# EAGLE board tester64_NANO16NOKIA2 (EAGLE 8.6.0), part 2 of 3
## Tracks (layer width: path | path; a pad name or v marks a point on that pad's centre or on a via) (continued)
+5V  (via drill 0.7, 0.7 pad 0.25) (continued)
  Top 0.61: U5.18 196.69,77.44 198.38,79.12 204,79.12 208.12,79.12 v209,79.25 | C7.2 U6.15 200.5,104.5 200,105 197.5,105 196.75,104.25 196.75,102.91 U6.18 | C7.2 209.48,102.85 v209.5,102.88 | U7.9 193.91,117.22 197.75,113.38 v206.88,113.38 | U7.18 196.44,130.94 196.5,131 199.12,131 | 199.12,131 203.75,131 206.75,131 v206.88,131.12 | U7.16 198.99,130.86 199.12,131 | U8.9 194.03,143.97 | U8.15 206.85,155.86 v207,156 | C7.2 | U6.9 194.16,92.09 196.98,89.26 v209.13,89.26 | v25,135.75 41.5,135.75 | 41.5,135.75 45.6,135.75 R86.2 | v41.25,138.25 41.25,136 41.5,135.75 | v29.75,108.75 29.75,109.75 31.5,111.5 34.24,111.5 C2.2 34.37,111.5 v38.5,111.5 39.5,112.5 R71.2 | v25.25,77 27.73,79.47 C6.2 29.02,79.5 v34.12,79.5 R55.2 | U5.9 194.16,63.09 v194.62,62.62 | R55.2 R54.2 R53.2 R52.2 R51.2 R50.2 R49.2 43.25,70.97 43.25,70 41.85,68.6 R48.2 R47.2 R46.2 R45.2 R44.2 R43.2 R42.2 R41.2 R40.2 | R55.2 R56.2 R57.2 R58.2 R59.2 R60.2 R61.2 R62.2 R63.2 R64.2 43.23,100.38 R65.2 R66.2 R67.2 R68.2 R69.2 R70.2 R71.2 | R33.2 R34.2 R35.2 R36.2 R37.2 R38.2 R39.2 R40.2 | R71.2 R72.2 R73.2 R74.2 R75.2 R76.2 R77.2 R78.2 R79.2 R80.2 R81.2 R82.2 R83.2 R84.2 R85.2 R86.2 | R86.2 R87.2 R88.2 R89.2 R90.2 R91.2 R92.2 R93.2 R94.2 R95.2 R96.2 v43.88,152 | v40.5,55.88 41.73,55.88 R40.2 | v215.5,89.25 212.25,89.25
  Top 0.813: v207,141.5 195.38,141.5 194.25,142.62 194.25,143.97 C4.2 | 199.45,46.25 R2.2 | U11.4 118.63,62.75 C44.+ 161,62.75 177.5,46.25 199.45,46.25 | U13.3 209.3,40.76 ARD1.J2.4 209.41,42.34 205.5,46.25 199.45,46.25 | 212.25,89.25 209.14,89.25 v209.13,89.26
  Bottom 0.406: U4.9 41.16,138.34 v41.25,138.25 | U1.18 U1.17 27.61,107.5 26.5,107.5 26,107 26,105.5 26.51,105 U1.15 | U2.18 21.93,49.43 21.62,49.12 21.62,46.88 | 21.62,46.88 21.62,46.12 22.25,45.5 22.9,45.5 U2.15 | U2.16 21.64,46.89 21.62,46.88 | 219.88,89.12 219.75,89.25
  Bottom 0.5: 36,55.88 33.62,53.5 33.62,52.75 32.84,51.97 U2.9 30.28,51.97 v30.5,52 | U2.18 24.93,49.43 v25.25,49.88
  Bottom 0.61: v207,156 v207,141.5 207,131.25 v206.88,131.12 v206.88,113.38 206.88,106 209.38,103.5 209.38,103 v209.5,102.88 209.38,102.88 208.66,102.16 208.66,90.28 209,89.94 v209.13,89.26 209,89.51 v209,79.25 209,72.12 203,66.12 203,62.62 | v25,135.75 25.75,135.75 25.8,135.81 U4.18 U4.17 U4.16 | U1.9 38.34,111.34 v38.5,111.5 | U1.18 29.7,108.81 v29.75,108.75 | U3.9 34.09,79.47 v34.12,79.5 | v25.25,77 23.09,77 U3.18 U3.17 | ARD1.J2.4 209.41,45.84 204.75,50.5 204.75,53.62 203,55.38 203,62.62 | v194.62,62.62 203,62.62 | 36,55.88 v40.5,55.88 | 220.75,80.5 220.75,88.25 219.88,89.12 | 219.75,89.25 v215.5,89.25
  Bottom 0.813: v43.88,152 43.88,170.5 56,182.62 203.38,182.62 206.88,179.12 206.88,156.12 v207,156 | 220.75,80.5 221.66,79.59 J22.3 J22.1 J22.2
A0
  Top 0.406: R103.2 R104.1 123.7,55.7 129,61 160,61 175.5,45.5 175.5,45.25 176,44.75 185.21,44.75 ARD1.J2.12
D0
  Top 0.61: SW6.2 150.75,43 161.5,32.25 161.5,21.25 164.5,18.25 208.75,18.25 214.5,24 ARD1.J1.2
  Bottom 0.61: SW6.2 SW6.1
D2  (via drill 0.7)
  Top 0.406: R106.1 85.25,64.5 v85.5,64.75
  Top 0.61: v85.5,68.75 159.25,68.75 v175.5,52.5
  Bottom 0.406: 85.5,65.25 v85.5,64.75 v85.5,68.75
  Bottom 0.61: v175.5,52.5 175.5,39.5 186.5,28.5 204,28.5 ARD1.J1.5
D11
  Top 0.61: SW3.2 SW3.1
  Bottom 0.406: SW3.1 176.05,15.55 184,23.5 ARD1.J1.14
D12
  Top 0.406: ARD1.J1.15 181.47,26.53 176.5,31.5 173.18,31.5 SW2.2
  Top 0.61: SW2.2 SW2.1
D13
  Top 0.406: SW1.1 176.8,35.8 181,40 181,40.4 ARD1.J2.15
  Top 0.61: SW1.2 SW1.1
DC.1
  Bottom 0.61: DIS1.J1.3 195.83,14.83 199,18 199,18.83 R138.1
DIN.1
  Bottom 0.61: DIS1.J1.4 198.37,14.62 202,18.25 R139.1
DSUB  (via drill 0.7)
  Top 0.406: v223.5,55.5 215.25,55.5 v215,55.75 | ARD1.J1.12 189.09,30.16 v189,30.25
  Bottom 0.406: J22.4 217.09,79.59 215,77.5 v215,55.75 | v189,30.25 222,30.25 223.75,32 223.75,55.25 v223.5,55.5
GND  (via drill 0.7, 0.7 pad 0.25)
  Top 0.406: C3.1 203.12,128.98 202.62,128.48 | v39.25,137 34.51,137 C1.1 | C8.1 203.62,77.88 203.75,78 | v34.62,50.75 35.5,50.75 35.62,50.62 36.12,50.62 36.38,50.38 36.25,50.25
  Top 0.5: C5.1 23.73,48.02 25.38,46.38
  Top 0.61: U6.10 195.43,92.2 197,90.62 v209.75,90.62 | v209.75,100.88 203.12,100.88 | 203.12,100.88 199.5,100.88 | 199.5,100.88 198.5,100.88 198,101.38 198,102.82 U6.17 | U6.16 199.24,101.14 199.5,100.88 | v210.12,78 203.75,78 199,78 197.97,76.97 U5.17 U5.16 U5.15 | v209.25,128.5 209.23,128.48 202.62,128.48 U7.15 200.25,127.25 199.62,126.62 198.38,126.62 197.72,127.28 U7.17 | U7.10 195.18,117.58 198,114.75 v209.25,114.75 | U8.10 195.3,144.68 C4.1 | C7.1 203.38,101.12 203.12,100.88 | C25.2 C26.2 C27.2 C28.2 C29.2 C30.2 C31.2 C32.2 | C33.2 C34.2 C35.2 C36.2 C37.2 C38.2 C39.2 C40.2 193.42,89.78 195.2,87.99 | v29.75,106.25 30,106.25 33.5,109.75 34.29,109.75 C2.1 34.54,109.5 v39,109.5 | v34.25,77.75 29.02,77.75 | 29.02,77.75 C6.1 | 29.02,77.75 28.5,77.75 v25.25,74.5 | R104.2 101.5,50.99 SW6.3 | C17.2 C18.2 C19.2 C20.2 C21.2 C22.2 C23.2 192.25,60.77 | 192.25,60.77 C24.2 | 192.28,60.75 192.25,60.77 | v30.5,50.62 29.5,50.62 v25.25,46.38
  Top 0.813: v209.25,142.88 197.1,142.88 C4.1 | C25.2 209.06,106.72 v209.25,106.53 | C1.1 23.63,137.13 23.25,136.75 | 23.25,131.5 v23.25,131.75 23.25,130.25 19.5,126.5 19.5,106.25 30,106.25 | ARD1.J1.4 209.3,25.74 U13.1 214.03,32.72 v214.25,32.5 | C44.- 125.5,67.5 112.75,67.5 110.95,65.7 U11.1 99.78,65.53 99.75,65.5 | Q2.2 71.55,53.3 | SW1.4 SW1.3 | U5.10 195.43,63.83 196.12,63.12 196.12,61 195.88,60.75 192.9,60.75 C24.2
  Top 1.016: 193.42,89.78 193.72,89.78 195.25,88.25 207.75,88.25 208.25,87.75 v210.12,87.75 | 99.75,65.5 92.25,65.5 90.5,67.25 77.3,67.25 | SW3.3 SW3.4 | SW2.4 SW2.3
  Bottom 0.406: U4.10 39.17,137.07 v39.25,137 | U2.10 34.58,50.7 v34.62,50.75
  Bottom 0.5: C47.- 207,4.12 208.62,5.75 208.62,7.16 JP1.3 | U4.15 26.74,132 26.5,131.75 v23.25,131.75 | U2.17 24.72,48.16 25.5,47.38 25.5,46.62 v25.25,46.38
  Bottom 0.61: v209.25,106.53 v209.25,114.75 v209.25,128.5 v209.25,142.88 | 209.25,105.52 209.25,105.12 211.12,103.25 211.12,102.25 v209.75,100.88 v209.75,90.62 210.12,90.25 v210.12,87.75 v210.12,78 210.25,77.88 | U1.16 29.73,106.27 v29.75,106.25 | U1.10 38.42,110.08 v39,109.5 | U3.10 33.8,78.2 v34.25,77.75 | v25.25,74.5 23.13,74.5 U3.16 U3.15 | U2.10 30.58,50.7 v30.5,50.62
  Bottom 0.813: v209.25,106.53 209.25,105.52 | R3.1 R4.1 75,6.92 R5.1 77.38,7.05 R6.1 79.88,7.17 R7.1 R8.1 R9.1 R10.1 R11.1 R12.1 R13.1 97.38,7.3 R14.1 R15.1 R16.1 R17.1 R18.1 R19.1 R20.1 115,7.17 R21.1 117.38,7.3 R22.1 R23.1 R24.1 R25.1 R26.1 R27.1 R28.1 R29.1 R30.1 R31.1 R32.1 R97.1 R98.1 164.43,7.17 169,11.75 169,39.2 SW1.4 | SW6.4 SW6.3 91.49,61 74.75,61 71.15,57.4 | v214.25,32.5 214.25,40.63 ARD1.J2.2
  Bottom 1.016: C41.- 55,10.75 | 55,10.75 55,9.5 57.75,6.75 68.45,6.75 R3.1 | U12.1 54.8,10.95 55,10.75 | v25.25,46.38 25.25,29.12 v25,28.88
  other vias: 23.25,137.25 25,131.75 21.5,137.25 177.5,43 183,43 209,14.75 211,14.75
  pour Top (isolate 0.813): 2.12,184 223.5,184 223.5,2.12 2.12,2.12
  pour Bottom (isolate 0.813): 1.5,183.5 224,183.5 224,1 1.5,1
IDC  (via drill 0.7)
  Top 0.406: v171.5,3.75 171.75,3.75 173.75,1.75 v187.5,1.75
  Bottom 0.305: U2.21 24.38,53.24 26.12,51.49 26.12,42.62 27.75,41 | RN1.1 41.65,49 39.38,49 39.12,48.75 39.12,42.88 37.25,41 29,41 28.25,40.25
  Bottom 0.406: 27.75,41 28.25,40.5 28.25,40.25 28.25,18 42,4.25 171,4.25 v171.5,3.75 | v187.5,1.75 187.5,7.25 188.75,8.5 188.75,19.5 191.75,22.5 191.75,25.51 ARD1.J1.11
N$2
  Bottom 0.305: U2.22 24.37,54.51 26.62,52.25 26.62,43.5 28.62,41.5 37,41.5 38.62,43.12 38.62,49.62 38.88,49.88 RN1.2
N$3
  Bottom 0.305: U2.23 24.72,55.78 25,55.5 25,54.62 27.12,52.5 27.12,43.75 28.88,42 36.75,42 38.12,43.38 38.12,50.5 38.38,50.75 41.65,50.75 RN1.3
N$4
  Bottom 0.305: U2.24 25.08,57.05 25.5,56.62 25.5,54.88 27.62,52.75 27.62,43.88 29,42.5 36.38,42.5 37.62,43.75 37.62,51.12 38,51.5 41.7,51.5 RN1.4
N$5
  Bottom 0.305: U2.25 25.8,58.32 26,58.12 26,55.12 28.12,53 28.12,44.12 29.25,43 36,43 37,44 37,51.88 37.38,52.25 41.7,52.25 RN1.5
N$6
  Bottom 0.305: U2.26 26.16,59.59 26.5,59.25 26.5,55.38 28.62,53.25 28.62,44.5 29.5,43.62 35.75,43.62 36.5,44.38 36.5,52.62 37,53.12 41.67,53.12 RN1.6
N$7
  Bottom 0.305: U2.27 26.64,60.86 27,60.5 27,55.88 29.12,53.75 29.12,44.88 29.88,44.12 35.25,44.12 36,44.88 36,53 37,54 41.6,54 RN1.7
N$8
  Bottom 0.305: U2.28 27.12,62.13 27.5,61.75 27.5,56.12 29.62,54 29.62,45.25 30.25,44.62 34.88,44.62 35.5,45.25 35.5,53.38 36.75,54.62 41.67,54.62 RN1.8
N$9
  Bottom 0.305: U3.21 23.88,80.74 26.5,78.12 26.5,70.62 28.75,68.38 36.62,68.38 39.62,71.38 39.75,71.38 43,74.62 43,75.22 RN3.1 43.02,75.25
N$10
  Bottom 0.305: U3.22 24.24,82.01 24.5,81.75 24.5,81 27.12,78.38 27.12,70.88 29.12,68.88 36.25,68.88 42.25,74.88 42.25,75.62 42.75,76.12 RN3.2
N$11
  Bottom 0.305: U3.23 24.72,83.28 25,83 25,81.38 27.62,78.75 27.62,71.25 29.5,69.38 35.75,69.38 41.62,75.25 41.62,76.12 42.5,77 43.02,77 RN3.3
N$12
  Bottom 0.305: U3.24 25.33,84.55 25.5,84.38 25.5,81.62 28.12,79 28.12,71.5 29.75,69.88 35.5,69.88 41,75.38 41,76.25 42.5,77.75 43.08,77.75 RN3.4
N$13
  Bottom 0.305: U3.25 25.68,85.82 26,85.5 26,81.88 28.75,79.12 28.75,71.75 30.12,70.38 35.12,70.38 40.38,75.62 40.38,76.62 42.25,78.5 43.08,78.5 RN3.5
N$14
  Bottom 0.305: U3.26 26.03,87.09 26.5,86.62 26.5,82.5 29.38,79.62 29.38,72 30.38,71 34.88,71 36.62,72.75 36.75,72.75 39.88,75.88 39.88,76.88 42.38,79.38 43.05,79.38 RN3.6
N$15
  Bottom 0.305: U3.27 26.77,88.36 27,88.12 27,82.75 29.88,79.88 29.88,72.25 30.62,71.5 34.62,71.5 39.25,76.12 39.25,77 42.38,80.12 RN3.7
N$16
  Bottom 0.305: U3.28 26.87,89.63 27.5,89 27.5,83.12 30.38,80.25 30.38,72.62 31,72 34.25,72 38.62,76.38 38.62,77.12 42.5,81 43.02,81 RN3.8
N$17
  Bottom 0.406: R3.2 68.62,15.5 X6.A1 71.75,18.62 71.75,19.75 88.75,36.75 106.75,36.75 123.45,53.45 RN9.9
N$18
  Bottom 0.305: R4.2 72.38,9.88 72.5,10 72.5,16.88 X6.A2
  Bottom 0.406: RN9.10 124.25,53 106.75,35.5 89.75,35.5 74.5,20.25 74.5,18.88 X6.A2
N$19
  Bottom 0.305: R5.2 75.12,11.25 75,11.38 75,16.88 X6.A3
  Bottom 0.406: RN9.11 125.05,52.8 106.25,34 90.5,34 77.25,20.75 77.25,20.25 76.75,19.75 76.75,18.62 X6.A3
N$20
  Bottom 0.305: R6.2 77.5,16.88 X6.A4
  Bottom 0.406: RN9.12 125.85,52.6 105.75,32.5 92,32.5 79.5,20 79.5,18.88 X6.A4
N$21
  Bottom 0.305: R7.2 80,16.88 X6.A5
  Bottom 0.406: RN9.13 126.65,52.4 105.5,31.25 93.25,31.25 82,20 82,18.88 X6.A5
N$22
  Bottom 0.305: R8.2 82.38,10 82.5,10.12 82.5,16.88 X6.A6
  Bottom 0.406: RN9.14 127.45,52.2 105.5,30.25 94.75,30.25 84.25,19.75 84.25,18.62 X6.A6
N$23
  Top 0.406: Q1.3 91.9,49.91 SW5.2 91.04,49.05 R105.1
  Top 0.813: SW5.1 91.49,38.76 95.5,34.75 137,34.75 BT1.2+
  Top 1.016: SW5.1 89,43 72.25,26.25 58.62,26.25 46.75,14.38 D2.C
  Bottom 0.61: SW5.1 SW5.2
N$25
  Top 1.016: J12.3 29.3,14.5 D2.A
N$26
  Bottom 0.305: R9.2 85,16.25 86.25,17.5 X6.A7
  Bottom 0.406: RN9.15 128.25,52 105.5,29.25 96.75,29.25 86.75,19.25 86.75,18.62 X6.A7
N$27
  Bottom 0.305: R10.2 87.38,10.38 87.5,10.5 87.5,15.62 88.5,16.62 88.5,17.88 X6.A8
  Bottom 0.406: RN9.16 129.05,52.05 129,52 129,51.75 105.75,28.5 97.75,28.5 89,19.75 89,18.38 X6.A8
N$28
  Bottom 0.305: U1.21 29.63,112.61 31.75,110.5 31.75,101.75 34,99.5 41.5,99.5 44.5,102.5 44.5,106.75 44.75,107 45.67,107 RN5.1
N$29
  Bottom 0.305: R16.2 102.5,16 103.62,17.12 103.62,18 X6.A14
  Bottom 0.406: RN10.14 138.07,52.58 106.25,20.75 105.5,20.75 104,19.25 104,18.38 X6.A14
N$30
  Bottom 0.305: U1.22 29.12,113.89 32.25,110.75 32.25,102.25 34.5,100 41.25,100 44,102.75 44,107.25 44.5,107.75 RN5.2
N$31
  Bottom 0.305: U1.23 29.09,115.16 29.5,114.75 29.5,114.25 33,110.75 33,102.5 34.75,100.75 41.25,100.75 43.5,103 43.5,108.25 43.75,108.5 45.67,108.5 RN5.3
N$32
  Bottom 0.305: U1.24 29.08,116.42 30,115.5 30,114.5 33.5,111 33.5,102.75 35,101.25 41,101.25 43,103.25 43,109 43.25,109.25 45.62,109.25 RN5.4
N$33
  Bottom 0.305: U1.25 29.8,117.69 30.5,117 30.5,114.75 34,111.25 34,103 35.25,101.75 40.75,101.75 42.5,103.5 42.5,109.75 43,110.25 45.62,110.25 RN5.5
N$34
  Bottom 0.305: U1.26 30.03,118.97 31,118 31,115.25 34.5,111.75 34.5,103.5 35.75,102.25 40.5,102.25 42,103.75 42,110.25 42.75,111 45.67,111 RN5.6
N$35
  Bottom 0.305: U1.27 31.27,120.23 31.5,120 31.5,115.5 35,112 35,103.75 36,102.75 40.25,102.75 41.5,104 41.5,111.75 RN5.7
N$36
  Bottom 0.305: U1.28 31.25,121.5 32,120.75 32,115.75 35.5,112.25 35.5,104 36.25,103.25 40,103.25 41,104.25 41,112 41.5,112.5 45.67,112.5 RN5.8
N$37
  Bottom 0.305: U4.21 28.38,139.62 31.75,136.25 31.75,129.25 34,127 39.75,127 44.75,132 45.67,132 RN7.1
N$38
  Bottom 0.305: U4.22 28.62,140.88 29,140.5 29,139.75 32.25,136.5 32.25,129.5 34.25,127.5 39.25,127.5 44.5,132.75 RN7.2
N$39
  Bottom 0.305: U4.23 28.84,142.16 29.5,141.5 29.5,140 32.75,136.75 32.75,129.75 34.5,128 39,128 43.75,132.75 43.75,133 44.25,133.5 45.67,133.5 RN7.3
N$40
  Bottom 0.305: U4.24 29.33,143.43 30,142.75 30,140.25 33.25,137 33.25,130 34.5,128.75 39,128.75 43.25,133 43.25,133.75 43.75,134.25 45.62,134.25 RN7.4
N$41
  Bottom 0.305: U4.25 29.55,144.69 30.5,143.75 30.5,140.5 33.75,137.25 33.75,130.25 34.75,129.25 38.75,129.25 42.75,133.25 42.75,134.75 43.25,135.25 45.62,135.25 RN7.5
N$42
  Bottom 0.305: U4.26 30.28,145.97 31,145.25 31,140.75 34.25,137.5 34.25,130.5 35,129.75 38.5,129.75 42.25,133.5 42.25,135.5 42.75,136 45.67,136 RN7.6
N$43
  Bottom 0.305: U4.27 30.77,147.24 31.5,146.5 31.5,141.25 34.75,138 34.75,131 35.5,130.25 38.25,130.25 41.75,133.75 41.75,136.25 42.25,136.75 RN7.7
N$44
  Bottom 0.305: U4.28 30.99,148.5 32,147.5 32,141.75 35.25,138.5 35.25,131.25 35.75,130.75 38,130.75 41.25,134 41.25,136.75 42,137.5 45.67,137.5 RN7.8
N$45
  Bottom 0.305: R12.2 92.5,16.12 93.38,17 93.38,17.75 X6.A10
  Bottom 0.406: RN10.10 134.88,53.38 107,25.5 100.25,25.5 94.25,19.5 94.25,18.62 X6.A10
N$46
  Bottom 0.305: R15.2 100,16.12 101.25,17.38 X6.A13
  Bottom 0.406: RN10.13 137.28,52.77 106.25,21.75 104.25,21.75 102,19.5 102,18.88 X6.A13
N$47
  Bottom 0.305: R13.2 95,16.12 96,17.12 96,17.88 X6.A11
  Bottom 0.406: RN10.11 135.68,53.17 106.75,24.25 101.5,24.25 96.5,19.25 96.5,18.38 X6.A11
N$48
  Bottom 0.305: R17.2 105,16.25 106.12,17.38 106.12,18 X6.A15
  Bottom 0.406: X6.A15 106.75,18.62 106.75,20.25 142.25,55.75 142.25,58.12 138.88,61.5 RN10.15
N$49
  Bottom 0.813: X2.A3 X2.A2 X2.A1 C41.+ 54.5,18 54.37,18.13 U12.4
N$50
  Bottom 0.305: R19.2 110,16.25 110.88,17.12 110.88,17.75 X6.A17
  Bottom 0.406: X6.A17 111.25,19 118.25,26 127,26 136,35 136,39.25 154.62,57.88 155.2,58.45 | 155.2,58.45 155.25,58.5 | RN11.9 155.2,58.45
N$51
  Bottom 0.305: R23.2 120,15.88 121.25,17.12 X6.A21
  Bottom 0.406: 121.5,18.38 X6.A21 122,18.88 122,19.75 124.5,22.25 128,22.25 158.4,52.65 RN11.13
N$52
  Bottom 0.305: R18.2 107.62,10 107.5,10.12 107.5,16.25 108.5,17.25 108.5,17.88 X6.A16
  Bottom 0.406: X6.A16 109,18.38 109,21.5 143,55.5 143,58.5 139.75,61.75 139.75,67.72 RN10.16
N$53
  Bottom 0.305: R25.2 124.88,10.12 125,10.25 125,16.88 X6.A23
  Bottom 0.406: RN11.15 160,52.25 128.25,20.5 127.75,20.5 126.25,19 X6.A23
N$54
  Bottom 0.305: R26.2 127.5,16.25 128.5,17.25 128.5,17.88 X6.A24
  Bottom 0.406: 128.62,18.25 X6.A24 129.25,18.62 129.25,20.5 160.8,52.05 RN11.16
N$55
  Bottom 0.305: R27.2 130,16 131,17 131,17.88 X6.A25
  Bottom 0.406: RN12.9 167.45,53.45 134.5,20.5 132.75,20.5 131.25,19 X6.A25
N$56
  Bottom 0.305: R28.2 132.5,16.25 133.5,17.25 133.5,17.88 X6.A26
  Bottom 0.406: RN12.10 168.25,53.25 134,19 134,18.38 X6.A26
N$58
  Bottom 0.305: R29.2 135.12,9.25 135,9.38 135,16 135.88,16.88 135.88,17.75 X6.A27
  Bottom 0.406: RN12.11 169.05,53.05 142.25,26.25 142.25,25.25 136.25,19.25 X6.A27
N$59
  Top 0.406: Q1.2 91.77,54.25 Q2.3 87.5,54.1 R105.2
N$60
  Bottom 0.305: R31.2 140,15.62 141.12,16.75 141.12,17.5 141.12,18 X6.A29
  Bottom 0.406: 141.12,18.25 X6.A29 | RN12.13 170.65,52.65 145.5,27.5 145.5,27.25 144.75,26.5 144.75,22.5 141.25,19 141.25,17.62 141.12,17.5
N$61
  Top 0.813: BT1.2- 67.45,38.2 75.5,46.25 129.2,46.25 BT1.1+
N$62  (via drill 0.8)
  Top 1.016: J12.1 17.62,7.75 16.25,6.38 11.88,6.38 9.38,8.88 9.38,14.38 12.12,17.12 12.25,17.12 14.12,19 47.75,19 56.88,28.12 63.12,28.12 v64.5,29.5
  Bottom 1.016: v64.5,29.5 64.5,54.45 BT1.1-
N$63
  Bottom 0.305: R11.2 90,15.75 90.62,16.38 90.62,17.5 X6.A9
  Bottom 0.406: RN10.9 134.07,53.58 107.5,27 99,27 91.5,19.5 91.5,18.38 X6.A9
N$64
  Bottom 0.61: R136.2 194.25,25.55 ARD1.J1.10
N$65
  Bottom 0.305: R30.2 137.5,16.38 138.38,17.25 138.38,17.75 X6.A28
  Bottom 0.406: 139,18.38 X6.A28 138.75,20 143.5,24.75 143.5,26.5 169.85,52.85 RN12.12
N$66
  Bottom 0.61: R137.2 196.75,25.59 ARD1.J1.9
N$67
  Bottom 0.305: R32.2 142.62,9.5 142.5,9.62 142.5,15.75 143.5,16.75 143.5,17.88 X6.A30
  Bottom 0.406: X6.A30 144.12,18.5 144,18.62 144,20.25 146.5,22.75 146.5,27.5 171.45,52.45 RN12.14
N$68
  Bottom 0.61: R138.2 ARD1.J1.8
N$69
  Bottom 0.61: R139.2 202,25.42 ARD1.J1.7
N$71
  Bottom 0.61: R140.2 204.75,25.21 ARD1.J1.6
N$72
  Top 0.5: DIS1.J1.7 JP1.2
N$81
  Bottom 0.305: R14.2 97.5,16.38 98.38,17.25 98.38,17.75 X6.A12
  Bottom 0.406: RN10.12 136.47,52.98 106.5,23 102.75,23 99.25,19.5 99.25,18.62 X6.A12
N$87
  Bottom 0.305: R20.2 112.5,15.75 113.62,16.88 113.62,18 X6.A18
  Bottom 0.406: RN11.10 156,57.75 137.25,39 137.25,35 127.25,25 119,25 114,20 114,18.38 X6.A18
N$88
  Bottom 0.305: R21.2 115.05,9.2 115,9.25 115,15.75 116.12,16.88 116.12,18 X6.A19
  Bottom 0.406: RN11.11 156.8,57 138.25,38.45 138.25,34.75 127.75,24.25 121.75,24.25 116.5,19 116.5,18.38 X6.A19
N$89
  Bottom 0.305: R22.2 117.5,16 118.62,17.12 118.62,18 X6.A20
  Bottom 0.406: RN11.12 157.6,52.85 128,23.25 123.25,23.25 119.25,19.25 119.25,18.62 X6.A20
N$91
  Bottom 0.305: R24.2 122.5,16.12 123.62,17.25 123.62,17.5 123.62,18 X6.A22
  Bottom 0.406: 123.88,17.75 123.62,17.5 | RN11.14 159.2,52.45 128.25,21.5 125.75,21.5 124.5,20.25 124.5,18.88 X6.A22
N$107
  Bottom 0.305: R97.2 145,16 146,17 146,17.88 X6.A31
  Bottom 0.406: 146.38,18.25 X6.A31 146.25,19.5 147.25,20.5 147.25,27 172.25,52 RN12.15
N$108
  Bottom 0.305: R98.2 147.5,16 148.5,17 148.5,17.88 X6.A32
  Bottom 0.406: 148.62,18.25 148.62,27.12 173,51.5 173,67.62 RN12.16
  Bottom 0.61: 148.62,18.25 X6.A32
N$112
  Top 0.813: U11.3 110.92,61 98.75,61 94.73,56.98 Q1.1 97.5,53.75 | 97.5,53.75 97.95,53.75 R103.1 | SW5.4 97.51,53.74 97.5,53.75
  Bottom 0.61: SW5.3 SW5.4
  Bottom 0.813: U12.3 43.55,10.95 40.5,14 40.5,19.5 45.25,24.25 74.25,24.25 90,40 94.51,40 SW5.3
N$114
  Top 0.406: Q2.1 85.15,57.2 R106.2
PA0_5
  Top 0.305: U5.21 192.88,73.38 189.12,69.62 179.5,69.62 172.62,76.5 164.81,76.5 J2.1 162.94,74.62 160.88,74.62 158.62,76.88 J4.1
  Top 0.406: U5.21 192.88,74.88 193.38,75.38 193.38,76.15 C9.1 | J6.1 142.92,76.12 J8.1 132.13,76.12 130.75,77.5 124.75,77.5 123.25,76 122.72,76 J10.1 122.33,76.25 121.5,76.25 120.5,77.25 118.12,77.25 115.5,79.88 115.5,171.5 119.49,175.49 J13.1 120.51,175.49 121.75,174.25 128.25,174.25 129.38,175.38 129.93,175.38 J15.1 130.94,175.56 132.12,174.38 138.75,174.38 139.5,175.12 140.62,175.12 J17.1 141.49,175.01 142.62,173.88 143.75,173.88 146.62,176.75 J19.1 152.38,176.75 153.75,175.38 162.4,175.38 J21.1
  Bottom 0.305: RN9.1 123.45,75.12 J10.1 | J6.1 152.27,74.9 J4.1
PA0_6
  Top 0.305: U6.21 192.88,102.84 192.88,102.5 188.75,98.38 167,98.38 165.38,96.75 164.75,96.75 J2.17 163.9,96.65 162.62,95.38 161.5,95.38 159.75,97.12 154.32,97.12 J4.17
  Top 0.406: C25.1 193.38,104.62 193,104.25 193,102.97 U6.21 | J15.17 125.11,155.24 123.75,153.88 121.03,153.88 J13.17 | J10.17 122.9,96.5 124,96.5 125.12,97.62 131.38,97.62 132.56,96.44 J8.17 142.92,96.44 J6.17
  Bottom 0.305: RN11.1 155.2,70.08 155.5,70.38 155.5,95.94 J4.17 154.18,97.12 153.38,97.12 152.12,95.88 151.12,95.88 150.47,95.22 J6.17
  Bottom 0.406: J13.17 119.73,155.14 121,153.88 122.75,153.88 127.88,148.75 127.88,124.12 128.88,123.12 128.88,101.38 124,96.5 122.9,96.5 J10.17
PA0_7
  Top 0.305: U7.21 192.62,127 190.25,124.62 187.5,124.62 179.84,116.97 J2.33 163.84,116.97 162.62,115.75 156.88,115.75 155.25,117.38 154.39,117.38 J4.33
  Top 0.406: J10.33 122.65,116.64 124,118 131.25,118 132.49,116.76 J8.33 142.92,116.76 J6.33
  Bottom 0.406: J6.33 150.53,115.53 151.12,116.12 152.86,116.12 J4.33
PA0_8
  Top 0.305: 179.38,150.75 179.5,150.75 180.38,151.62 188.5,151.62 188.88,152 189.62,152 192.76,155.13 192.76,155.26 | J2.49 163.92,137.29 162.75,136.12 156.75,136.12 155.25,137.62 154.46,137.62 J4.49 153.33,137.83 152.12,136.62 144.92,136.62 J6.49
  Top 0.406: U8.21 192.76,155.26 | 179.38,150.75 166.12,137.5 164.86,137.5 J2.49
PA1_5
  Top 0.305: U5.22 191.62,73.37 188.38,70.12 179.88,70.12 172.25,77.75 163.53,77.75 J2.2 162.06,76.38 160.62,76.38 158.88,78.12 153.12,78.12 151.88,76.88 J4.2
  Top 0.406: C10.1 192.12,75.88 191.62,75.38 U5.22 | J6.2 141.46,74.75 132.25,74.75 130.88,76.12 J8.2 130.11,75.75 124.5,75.75 123.5,74.75 121.25,74.75 120.1,75.9 J10.2 120.03,76 117.88,76 114.88,79 114.88,173.5 118.25,176.88 120.88,176.88 J13.2 122.74,175.49 124.12,176.88 131.32,176.88 J15.2 132.68,175.56 134,176.88 141.38,176.88 142.88,175.38 142.91,175.38 J17.2 143.39,175.01 146.38,178 153.39,178 J19.2 155.12,176.75 156.25,177.88 163.1,177.88 J21.2
  Bottom 0.305: RN9.2 124.25,76 123,77.25 121.42,77.25 J10.2 | J6.2 141.61,75.1 142.62,76.12 150.38,76.12 151.12,76.88 J4.2
PA1_6
  Top 0.305: 164.12,97.88 165.62,97.88 166.62,98.88 188.38,98.88 191.62,102.12 191.62,102.84 U6.22 | J2.18 161.6,96.65 159.75,98.5 153.01,98.5 J4.18
  Top 0.406: 164.12,97.88 163.33,97.88 J2.18 | U6.22 191.62,104.12 191.75,104.25 191.75,104.9 C26.1 | J15.18 132.26,155.24 131,156.5 125.25,156.5 123.88,155.12 122.31,155.12 J13.18 | J10.18 120.25,96.25 121.5,95 123.88,95 125.5,96.62 130.3,96.62 J8.18 131.06,96.44 132.25,95.25 141.57,95.25 J6.18
  Bottom 0.305: RN11.2 156,97.75 155.25,98.5 153.01,98.5 J4.18 151.64,97.12 151.12,97.12 150.5,96.5 142.88,96.5 J6.18 | 129.38,123.88 129.38,97.55
  Bottom 0.406: 129.38,123.88 128.5,124.75 128.5,149.38 123,154.88 122.56,154.88 J13.18 | 129.38,97.55 J8.18
PA1_7
  Top 0.305: J2.34 162.97,116.97 164.12,118.12 180.25,118.12 187.25,125.12 189.75,125.12 191.38,126.75 U7.22 | 162.01,116.88 157,116.88 155.12,118.75 153.62,118.75 152.38,117.5 151.72,117.5 J4.34
  Top 0.406: 162.01,116.88 J2.34 | J10.34 120.1,116.39 121.25,115.25 123.25,115.25 124.5,116.5 130.22,116.5 J8.34 130.99,116.76 132.25,115.5 141.57,115.5 J6.34
  Bottom 0.406: J6.34 142.16,115.53 143.5,116.88 151.07,116.88 J4.34
PA1_8
  Top 0.305: 178.5,151.38 179.25,152.12 188.12,152.12 188.5,152.5 189.12,152.5 191.49,154.87 191.49,155.12 | J2.50 156.71,137.29 154.88,139.12 153,139.12 J4.50 143.58,137.83 J6.50
  Top 0.406: U8.22 191.49,155.12 | 178.5,151.38 165.75,138.62 164.38,138.62 163.04,137.29 J2.50
PA2_5
  Top 0.305: U5.23 190.34,73.34 187.62,70.62 180.12,70.62 172,78.75 164.76,78.75 J2.3 164.4,78.62 163.5,78.62 162.62,77.75 160.88,77.75 159.21,79.41 J4.3
  Top 0.406: C11.1 190.75,75.75 190.38,75.38 190.38,74.01 U5.23 | J6.3 144.08,77.5 143.75,77.5 142.59,78.66 J8.3 132.34,78.66 131,80 124.75,80 123.25,78.5 122.67,78.5 J10.3 121.78,78.47 120.5,79.75 118.88,79.75 116.75,81.88 116.75,170.38 119.33,172.95 J13.3 120.42,172.95 121.62,171.75 128.25,171.75 129.38,172.88 129.97,172.88 J15.3 130.61,173.01 131.88,171.75 139.25,171.75 140.12,172.62 140.58,172.62 J17.3 141.03,172.47 142.25,171.25 144,171.25 146.88,174.12 152.03,174.12 J19.3 152.17,174.21 153.38,173 162.56,173 J21.3
  Bottom 0.305: RN9.3 125.05,76.45 123.25,78.25 122.87,78.25 J10.3 | J6.3 150.19,77.44 150.88,78.12 152.96,78.12 J4.3
PA2_6
  Top 0.305: U6.23 190.38,102.83 190.38,102.25 187.5,99.38 164.83,99.38 J2.19 163.69,99.19 162.5,98 161.12,98 159.25,99.88 154.39,99.88 J4.19
  Top 0.406: U6.23 190.34,104.87 C27.1 | J15.19 124.69,152.69 123.5,151.5 120.86,151.5 J13.19 | J10.19 122.85,99 124.25,99 125.5,100.25 131,100.25 132.27,98.98 J8.19 142.92,98.98 J6.19
  Bottom 0.305: RN11.3 156.8,98.95 156,99.75 154.26,99.75 J4.19 154.24,99.75 153.38,99.75 151.88,98.25 151.12,98.25 150.63,97.75 J6.19
  Bottom 0.406: J13.19 120.12,152.63 121.38,151.38 122.75,151.38 126.5,147.62 126.5,123.62 127.62,122.5 127.62,102.25 124.16,98.79 J10.19
PA2_7
  Top 0.305: U7.23 190.12,128.45 190.12,126.38 189.38,125.62 187,125.62 180.88,119.51 J2.35 164.26,119.51 163.12,118.38 156.38,118.38 154.75,120 154.31,120 J4.35
  Top 0.406: J8.35 142.92,119.3 J6.35
  Bottom 0.406: J6.35 150.57,118.08 151.38,118.88 153.07,118.88 J4.35
PA2_8
  Top 0.305: 178,152 178.12,152 178.75,152.62 187.88,152.62 188.25,153 188.5,153 190.22,154.72 U8.23 | J2.51 164.45,139.83 163.25,138.62 156.62,138.62 154.88,140.38 J4.51
  Top 0.406: 178,152 165.88,139.88 164.69,139.88 J2.51
PA3_5
  Top 0.305: U5.24 189.07,73.33 186.88,71.12 180.38,71.12 171.38,80.12 163.36,80.12 J2.4 161.97,79 160.88,79 159.12,80.75 153.12,80.75 151.79,79.41 J4.4
  Top 0.406: C12.1 189.38,75.62 189.12,75.38 189.12,74.03 U5.24 | J6.4 141.54,77.5 132.25,77.5 131.09,78.66 J8.4 124.66,78.66 123.25,77.25 121.75,77.25 120.5,78.5 120.1,78.5 J10.4 120.08,78.5 118.88,78.5 116.12,81.25 116.12,170.88 119.5,174.25 120.62,174.25 121.92,172.95 J13.4 128.2,172.95 129.5,174.25 130.62,174.25 131.86,173.01 J15.4 139.39,173.01 140.12,173.75 141.25,173.75 142.5,172.5 143.25,172.5 J17.4 143.97,172.47 147,175.5 152.62,175.5 153,175.12 153,175 153.75,174.25 | 153.62,174.25 153.75,174.25 | 153.75,174.25 154.6,174.25 J19.4 161.95,174.21 162.25,174.5 163.94,174.5 J21.4
  Bottom 0.305: RN9.4 125.85,77.15 123.25,79.75 121.38,79.75 J10.4 | J6.4 141.61,77.6 142.75,78.75 151.05,78.75 J4.4
PA3_6
  Top 0.305: 164.25,100.5 165.25,100.5 165.88,99.88 186.62,99.88 189.12,102.38 189.12,102.81 U6.24 | J2.20 160.94,99.19 159,101.12 153.1,101.12 J4.20
  Top 0.406: 164.25,100.5 163.42,100.5 J2.20 | U6.24 189.07,104.97 C28.1 | J15.20 132.31,152.69 131,154 125.12,154 124.12,153 122.64,153 J13.20 | J10.20 121.4,97.5 123.75,97.5 125.23,98.98 J8.20 131.02,98.98 132.25,97.75 J6.20
  Bottom 0.305: RN11.4 157.6,99.28 155.75,101.12 153.1,101.12 J4.20
  Bottom 0.406: J13.20 122.62,152.63 127.12,148.12 127.12,123.88 128.25,122.75 128.25,101.88 123.88,97.5 121.4,97.5 J10.20 | J6.20 141.75,97.75 143,99 150.97,99 J4.20
PA3_7
  Top 0.305: J2.36 163.01,119.51 164.25,120.75 181.38,120.75 186.75,126.12 188.5,126.12 188.88,126.5 188.88,128.43 U7.24 | 161.97,119.38 156.5,119.38 154.62,121.25 152.91,121.25 J4.36
  Top 0.406: 161.97,119.38 J2.36 | J8.36 131.2,119.3 132.5,118 141.53,118 J6.36
  Bottom 0.406: J6.36 141.61,118.11 142.88,119.38 150.38,119.38 151,120 151.66,120 J4.36
PA3_8
  Top 0.305: 177,152.62 177.5,153.12 187.75,153.12 189,154.38 189,155.81 U8.24 | J2.52 156.8,139.83 155,141.62 152.96,141.62 J4.52
  Top 0.406: U8.24 188.95,155.07 | 177,152.62 165.62,141.25 163.75,141.25 162.62,140.12 162.4,140.12 J2.52
PA4_5
  Top 0.305: U5.25 187.81,73.06 186.38,71.62 180.62,71.62 171.12,81.12 164.93,81.12 J2.5 164.49,81.25 163.62,81.25 162.5,80.12 161.12,80.12 159.3,81.95 J4.5 | 120.75,82.25 119.12,82.25 118.38,83
  Top 0.406: C13.1 188,75.25 187.75,75 187.75,74.03 U5.25 | 118.38,83 118.38,169.06 J13.5 119.84,170.41 121.12,169.12 127.75,169.12 129,170.38 130,170.38 J15.5 130.65,170.47 131.88,169.25 140.05,169.25 J17.5 141.06,169.94 142.38,168.62 144.62,168.62 147.75,171.75 152.02,171.75 J19.5 152.71,171.66 154,170.38 162.48,170.38 J21.5 162.61,170.5 | 120.75,82.25 121.99,81.01 J10.5 123.5,81 125,82.5 131.25,82.5 132.55,81.2 J8.5 142.05,81.2 143.25,80 144.12,80 J6.5
  Bottom 0.305: RN9.5 126.65,77 126.62,77.03 126.62,78 123.62,81.01 J10.5 | J6.5 150.35,79.97 151,80.62 152.92,80.62 J4.5
PA4_6
  Top 0.305: 187.88,102.78 U6.25 187.75,102.8 187.75,101.75 186.38,100.38 166.75,100.38 165.39,101.73 J2.21 163.73,101.73 162.5,100.5 160.62,100.5 158.88,102.25 154.28,102.25 J4.21
  Top 0.406: U6.25 187.81,104.97 C29.1 | J10.21 122.72,101.25 124,101.25 125.5,102.75 131,102.75 132.23,101.52 J8.21 142.92,101.52 J6.21
  Bottom 0.305: RN11.5 158.4,99.72 155.88,102.25 154.28,102.25 J4.21 | 150.88,100.75 151,100.75 151.12,100.88 152,100.88 152.75,101.62 152.75,101.75 153,102 153.38,102
  Bottom 0.406: J13.21 119.73,149.64 120.5,148.88 122.75,148.88 125.12,146.5 125.12,122.75 126.38,121.5 126.38,104 123.75,101.38 122.69,101.38 J10.21 | J6.21 150.42,100.3 150.88,100.75 | 153.38,102 153.97,102 J4.21
PA4_7
  Top 0.305: U7.25 187.5,128.43 187.5,126.88 187.25,126.62 186.5,126.62 181.93,122.05 J2.37 164.43,122.05 163.25,120.88 155.97,120.88 J4.37
  Top 0.406: J8.37 142.92,121.84 J6.37
  Bottom 0.406: J6.37 150.62,120.61 151.12,121.12 151.25,121.12 151.5,121.38 153.03,121.38 J4.37
PA4_8
  Top 0.305: 176.62,153.25 177,153.62 186.38,153.62 187.75,155 187.75,155.11 187.68,155.18 | J2.53 163.87,142.37 162.75,141.25 156.38,141.25 154.75,142.88 154.29,142.88 J4.53
  Top 0.406: U8.25 187.68,155.18 | 176.62,153.25 166.25,142.88 165.15,142.88 J2.53
PA5_5
  Top 0.305: U5.26 186.53,73.53 185.12,72.12 180.88,72.12 170.25,82.75 163.44,82.75 J2.6 161.89,81.62 161,81.62 159.38,83.25 153.25,83.25 151.95,81.95 J4.6
  Top 0.406: C14.1 186.62,74.07 U5.26 | J6.6 141.58,80 132.25,80 131.05,81.2 J8.6 124.7,81.2 123.25,79.75 122,79.75 120.75,81 120.12,81 J10.6 119.99,81.12 119.25,81.12 117.5,82.88 117.5,169.88 119.12,171.5 120.5,171.5 121.59,170.41 J13.6 127.91,170.41 129.25,171.75 130.88,171.75 132.12,170.5 132.62,170.5 J15.6 139.47,170.47 140.25,171.25 141.12,171.25 142.44,169.94 J17.6 144.81,169.94 147.75,172.88 152.62,172.88 153.38,172.12 154.19,172.12 J19.6 161.79,171.66 162,171.88 164.02,171.88 J21.6
  Bottom 0.305: RN9.6 127.45,78.8 123.88,82.38 121.47,82.38 J10.6 | J6.6 142.75,81.12 150.25,81.12 151.12,82 151.67,82 J4.6
PA5_6
  Top 0.305: 164.25,103 165.25,103 167.38,100.88 185.75,100.88 186.5,101.62 186.5,102.82 U6.26 | J2.22 160.39,101.73 158.62,103.5 152.94,103.5 J4.22
  Top 0.406: 164.25,103 163.38,103 J2.22 | C30.1 186.38,103.02 U6.26 | J10.22 121.44,100 124,100 125.52,101.52 J8.22 131.23,101.52 132.5,100.25 141.56,100.25 J6.22
  Bottom 0.305: RN11.6 159.2,101.05 156.75,103.5 152.94,103.5 J4.22
  Bottom 0.406: J13.22 122.53,150.09 125.75,146.88 125.75,123.12 127,121.88 127,102.62 124.5,100.12 121.38,100.12 120.17,101.33 J10.22 | J6.22 141.61,100.48 142.62,101.5 150.94,101.5 J4.22
PA5_7
  Top 0.305: U7.26 186.25,128.44 186.25,127.25 182.38,123.38 164.12,123.38 162.8,122.05 J2.38 156.95,122.05 155.12,123.88 152.99,123.88 J4.38
  Top 0.406: J8.38 130.48,121.77 131.75,120.5 141.49,120.5 J6.38
  Bottom 0.406: J6.38 142.88,121.88 150.99,121.88 J4.38
PA5_8
  Top 0.305: 175.88,153.88 176.12,154.12 185.25,154.12 186.19,155.07 186.5,155.07 186.41,155.16 | J2.54 156.5,142.37 154.75,144.12 152.92,144.12 J4.54
  Top 0.406: U8.26 186.41,155.16 | 175.88,153.88 165.75,143.75 163.49,143.75 J2.54
PA6_5
  Top 0.305: U5.27 185.26,73.27 184.62,72.62 181.12,72.62 169.88,83.88 164.72,83.88 J2.7 164.57,83.88 163.62,83.88 162.5,82.75 161,82.75 159.25,84.5 J4.7
  Top 0.406: C15.1 185.25,74 U5.27 | J10.7 122.84,83.75 123.75,83.75 125,85 131.25,85 132.51,83.74 J8.7 142.51,83.74 143.5,82.75 143.91,82.75 J6.7 | J13.7 119.73,167.77 120.88,166.62 127.88,166.62 129,167.75 129.92,167.75 J15.7 130.44,167.94 131.62,166.75 139.25,166.75 139.88,167.38 140.71,167.38 J17.7 141.36,167.39 142.5,166.25 145.75,166.25 148.62,169.12 J19.7 153,169.12 154.12,168 162.64,168 J21.7
  Bottom 0.305: RN9.7 128.25,81.38 126.12,83.5 122.69,83.5 J10.7 121.44,84.75 119.25,84.75 114.25,89.75 114.25,162.5 119.62,167.87 J13.7 | J6.7 150.76,82.52 151.5,83.25 153,83.25 J4.7
PA6_6
  Top 0.305: U6.27 185.25,102.84 185.25,101.88 184.75,101.38 168,101.38 165.11,104.27 J2.23 163.77,104.27 162.62,103.12 160.25,103.12 158.38,105 154.44,105 J4.23
  Top 0.406: C31.1 185,104.25 185.25,104 185.25,102.87 U6.27 | J10.23 122.77,103.75 124,103.75 125.5,105.25 131.25,105.25 132.44,104.06 J8.23 142.44,104.06 143.5,103 143.98,103 J6.23
  Bottom 0.305: RN11.7 160,102.62 157.88,104.75 154.31,104.75 J4.23
  Bottom 0.406: J13.23 119.73,147.39 121,146.12 122.88,146.12 123.75,145.25 123.75,122 125.12,120.62 125.12,105.5 123.5,103.88 J10.23 | J6.23 150.71,102.84 151.62,103.75 152.25,103.75 153,104.5 153.94,104.5 J4.23
PA6_7
  Top 0.305: U7.27 185,128.47 185,127.25 182.34,124.59 J2.39 164.22,124.59 163,123.38 156.75,123.38 155,125.12 J4.39
  Top 0.406: J8.39 142.92,124.38 J6.39
  Bottom 0.305: J6.39 150.66,123.16 151.5,124 153.12,124 J4.39
PA6_8
  Top 0.305: 175,154.5 175.12,154.62 184.75,154.62 185.12,155 185.12,155.84 U8.27 | J2.55 163.78,144.91 162.5,143.62 156.08,143.62 J4.55
  Top 0.406: J2.55 164.74,145 165.5,145 175,154.5
PA7_5
  Top 0.305: U5.28 180.77,73.98 169.62,85.12 163.28,85.12 J2.8 162.06,84 160.88,84 159.12,85.75 153.5,85.75 152.25,84.5 J4.8
  Top 0.406: C16.1 183.75,75.12 184.12,74.75 184.12,74.11 U5.28 | J10.8 120.95,83.55 122.25,82.25 123.5,82.25 125,83.75 J8.8 131.01,83.74 132.25,82.5 141.59,82.5 J6.8 | J13.8 127.87,167.87 129.25,169.25 130.62,169.25 132,167.88 132.58,167.88 J15.8 139.56,167.94 140.38,168.75 141,168.75 142.36,167.39 J17.8 144.89,167.39 148,170.5 152.62,170.5 153.88,169.25 154.52,169.25 J19.8 162,169.12 162.25,169.38 163.98,169.38 J21.8
  Bottom 0.305: RN9.8 129.05,82.31 J8.8 | J10.8 119.45,83.55 113.75,89.25 113.75,163.75 119.12,169.12 121.02,169.12 J13.8 | J6.8 141.64,82.52 142.88,83.75 150.97,83.75 J4.8
PA7_6
  Top 0.305: U6.28 168.02,102.85 165.38,105.5 163.62,105.5 | J4.24 151.71,104.84 152.88,106 158.25,106 159.88,104.38 162,104.38 J2.24
  Top 0.406: 163.62,105.5 163.33,105.5 J2.24 | C32.1 183.62,104 184,103.62 U6.28 | J10.24 121.35,102.62 124.12,102.62 125.5,104 130.42,104 J8.24 130.94,104.06 132.25,102.75 141.52,102.75 J6.24
  Bottom 0.305: RN11.8 160.8,102.97 J2.24
  Bottom 0.406: J13.24 122.7,147.55 124.5,145.75 124.5,122.12 125.75,120.88 125.75,105 123.38,102.62 121.35,102.62 J10.24 | J6.24 141.71,102.84 143,104.12 151.02,104.12 J4.24
PA7_7
  Top 0.305: U7.28 183.75,127 182.5,125.75 164,125.75 162.84,124.59 J2.40 157.53,124.59 155.75,126.38 153.75,126.38 152.5,125.12
  Top 0.406: J8.40 130.87,124.38 132,123.25 141.51,123.25 J6.40 | 152.5,125.12 J4.40
  Bottom 0.305: 145.38,125.12 144.62,124.38 142.82,124.38 J6.40
  Bottom 0.406: 145.38,125.12 J4.40
PA7_8
  Top 0.305: J2.56 157.34,144.91 155.5,146.75 153,146.75 J4.56
  Top 0.406: U8.28 175.36,155.86 165.62,146.12 163.32,146.12 J2.56
PB0_1
  Bottom 0.305: U2.1 33.37,62.13 36.5,59 41.8,59 RN2.1
PB0_2
  Bottom 0.305: U3.1 34.37,89.63 38.38,85.62 42.9,85.62 RN4.1
PB0_3
  Bottom 0.305: U1.1 38.25,121.5 42.25,117.5 45.9,117.5 RN6.1
PB0_4
  Bottom 0.305: U4.1 40,148.5 44.5,144 45.42,144 RN8.1
PB0_5
  Top 0.305: U5.1 184,65.87 186,67.88 188.38,67.88 193,72.5 209.38,72.5 212.38,75.5 212.38,82.25 212,82.62 181.5,82.62 177.5,86.62 164.78,86.62 J2.9 164.53,86.38 163.75,86.38 162.62,85.25 161,85.25 159.22,87.03 J4.9
  Top 0.406: U5.1 184,62.72 C17.1 | J10.9 122.81,86.25 123.5,86.25 124.75,87.5 131.25,87.5 132.47,86.28 J8.9 133.05,86.25 142.5,86.25 143.69,85.06 J6.9 | J13.9 119.8,165.33 121.12,164 127.88,164 129,165.12 129.83,165.12 J15.9 130.61,165.39 131.88,164.12 139.62,164.12 140.36,164.86 J17.9 141.02,164.86 142.25,163.62 146.5,163.62 149.38,166.5 152.02,166.5 J19.9 152.67,166.58 153.88,165.38 162.56,165.38 J21.9
  Bottom 0.305: RN10.1 134.07,69.7 134.5,70.12 134.5,84.8 J8.9 | J13.9 119.58,165.33 115.25,161 115.25,91.25 119.12,87.38 121.36,87.38 J10.9 | J6.9 150.56,85.06 151.25,85.75 152.88,85.75 153.5,86.38 153.59,86.38 J4.9
PB0_6
  Top 0.305: U6.1 184,94.12 187,97.12 189.38,97.12 190.75,98.5 211,98.5 212.5,100 212.5,107 211.25,108.25 166.88,108.25 165.38,106.75 164.7,106.75 J2.25 163.81,106.81 162.5,105.5 159.62,105.5 158.12,107 154.61,107 J4.25
  Top 0.406: C33.1 183.62,93.28 U6.1 | J10.25 122.73,106.5 123.5,106.5 124.75,107.75 131,107.75 132.15,106.6 J8.25 142.92,106.6 J6.25
  Bottom 0.305: RN12.1 167.45,106.17 166.62,107 164.83,107 J2.25
  Bottom 0.406: J13.25 119.73,124.14 123.88,120 123.88,107.64 J10.25 | J6.25 150.62,105.38 151.38,106.12 153.02,106.12 J4.25
PB0_7
  Top 0.305: U7.1 183.88,119.4 183.88,120 188,124.12 206.88,124.12 212.25,129.5 212.25,133 209.5,135.75 173.62,135.75 165,127.13 J2.41 164.13,127.13 163,126 157.25,126 155.62,127.62 154.3,127.62 J4.41 154.2,127.62 153.75,127.62 152.5,126.38 151.25,126.38 150.57,125.69 J6.41
PB0_8
  Top 0.305: 209.12,151.75 208.88,151.5 189.12,151.5 186.12,148.5 184.88,148.5 183.88,147.5 U8.1 | J2.57 163.7,147.45 162.62,146.38 157.12,146.38 155.5,148 J4.57
  Top 0.406: J2.57 165.32,147.45 177.12,159.25 210,159.25 211.75,157.5 211.75,154.38 209.12,151.75
PB1_1
  Bottom 0.305: U2.2 31.39,60.86 31,61.25 31,62.75 31.12,62.88 33.75,62.88 36.88,59.75 RN2.2
PB1_2
  Bottom 0.305: U3.2 31.27,88.36 31,88.62 31,90.25 31.12,90.38 34.38,90.38 38.38,86.38 42.85,86.38 RN4.2
PB1_3
  Bottom 0.305: U1.2 35.77,120.23 35.5,120.5 35.5,122.75 38,122.75 42.25,118.5 45.85,118.5 RN6.2
PB1_4
  Bottom 0.305: RN8.2 44.5,144.75 38,151.25 36,151.25 35.5,150.75 35.5,147.75 36.02,147.24 U4.2
PB1_5
  Top 0.305: U5.2 185.26,65.39 187.25,67.38 188.75,67.38 193.38,72 209.62,72 213.12,75.5 213.12,82.38 212.25,83.25 181.62,83.25 177.25,87.62 163.24,87.62 J2.10 161.97,86.62 160.88,86.62 159.25,88.25 153.62,88.25 152.41,87.03 J4.10
  Top 0.406: U5.2 185.26,62.74 C18.1 | J10.10 120.1,85.65 120.75,85 123.75,85 125,86.25 130.45,86.25 J8.10 130.51,86.25 131,86.25 132.19,85.06 J6.10 | J13.10 127.83,165.33 129.12,166.62 130.5,166.62 131.5,165.62 132.42,165.62 J15.10 139.52,165.39 140.12,166 141.5,166 142.64,164.86 J17.10 146.11,164.86 149.12,167.88 153.38,167.88 154.12,167.12 154.12,167.11 J19.10 161.96,166.58 162.12,166.75 164.06,166.75 J21.10
  Bottom 0.305: RN10.2 134.88,69.62 135.12,69.88 135.12,85.88 133.5,87.5 131.7,87.5 J8.10 | J10.10 119.28,86.09 114.75,90.62 114.75,162.12 119.25,166.62 120.97,166.62 J13.10 | J6.10 141.61,85.35 142.62,86.38 151.05,86.38 J4.10
PB1_6
  Top 0.305: U6.2 185.26,94.02 187.88,96.62 189.62,96.62 191,98 211.25,98 213.12,99.88 213.12,107.75 212.12,108.75 166.12,108.75 165.38,108 164,108 | J2.26 159.94,106.81 159.25,107.5 156.12,107.5 155,108.62 152.98,108.62 J4.26
  Top 0.406: 164,108 163,107 162.3,107 J2.26 | C34.1 185.12,93.5 U6.2 | J10.26 121.27,105.25 124.5,105.25 125.85,106.6 J8.26 130.9,106.6 132.25,105.25 141.48,105.25 J6.26
  Bottom 0.305: RN12.2 168.25,106.62 166.75,108.12 163.42,108.12 J2.26
  Bottom 0.406: J13.26 122.27,122.48 124.5,120.25 124.5,106.12 123.62,105.25 121.27,105.25 J10.26 | J6.26 141.61,105.48 142.75,106.62 150.98,106.62 J4.26
PB1_7
  Top 0.305: U7.2 185,119.28 185,119.75 185.25,120 185.25,120.12 188.75,123.62 207.25,123.62 212.75,129.12 212.75,133.38 209.62,136.5 173.38,136.5 165.25,128.38 164.38,128.38 163.13,127.13 J2.42 157.25,127.13 155.5,128.88 153.5,128.88 152.5,127.88 151.91,127.88 J4.42 151.03,127 143,127 141.69,125.69 J6.42
PB1_8
  Top 0.305: U8.2 185.14,147.14 186,148 186.38,148 189.38,151 210,151 210.38,151.38 | J2.58 157.55,147.45 155.62,149.38 153.09,149.38 J4.58
  Top 0.406: 210.38,151.38 212.5,153.5 212.5,158 210.5,160 176.62,160 165.38,148.75 163.41,148.75 J2.58
PB2_1
  Bottom 0.305: U2.3 31.41,59.59 30.5,60.5 30.5,62.88 31,63.38 34,63.38 36.88,60.5 41.8,60.5 RN2.3
PB2_2
  Bottom 0.305: U3.3 31.29,87.09 30.5,87.88 30.5,90.38 31,90.88 34.62,90.88 38.25,87.25 42.92,87.25 RN4.3
PB2_3
  Bottom 0.305: U1.3 35.78,118.97 35,119.75 35,123 35.25,123.25 38.25,123.25 42.33,119.17 RN6.3
PB2_4
  Bottom 0.305: RN8.3 45.42,145.5 44.75,145.5 38.5,151.75 35.75,151.75 35,151 35,147.25 36.25,146 36.82,146 U4.3
PB2_5
  Top 0.305: U5.3 186.53,65.41 188,66.88 189,66.88 193.62,71.5 210,71.5 213.88,75.38 213.88,82.38 212.38,83.88 182,83.88 176.88,89 164.68,89 J2.11 164.49,88.88 163.62,88.88 162.5,87.75 160.88,87.75 159.05,89.58 J4.11
  Top 0.406: U5.3 186.5,64.73 186.5,63.12 186.25,62.88 C19.1 | J10.11 122.77,88.75 123.5,88.75 124.75,90 131.25,90 132.43,88.82 J8.11 133.2,89 142.25,89 143.66,87.59 J6.11 | J13.11 119.84,162.79 121.12,161.5 124.62,161.5 125.75,162.62 129.88,162.62 J15.11 131.02,162.86 132.25,161.62 140.04,161.62 J17.11 141.19,162.31 142.38,161.12 147.38,161.12 150.12,163.88 151.94,163.88 J19.11
  Bottom 0.305: RN10.3 135.68,87.2 134.12,88.75 133.09,88.75 J8.11 | J13.11 119.29,162.79 116.25,159.75 116.25,93 119.25,90 121.28,90 J10.11 | J6.11 150.34,87.59 151,88.25 152.12,88.25 153.38,89.5 154.18,89.5 J4.11
PB2_6
  Top 0.305: U6.3 186.53,94.03 188.62,96.12 189.88,96.12 191.25,97.5 211.62,97.5 213.75,99.62 213.75,108.12 212.53,109.35 J2.27 163.85,109.35 162.5,108 157.25,108 155.38,109.88 154.27,109.88 J4.27
  Top 0.406: C35.1 186.38,93.48 U6.3 | J10.27 122.95,108.95 124.5,110.5 131,110.5 132.36,109.14 J8.27 142.92,109.14 J6.27
  Bottom 0.305: RN12.3 169.05,107.92 167.62,109.35 J2.27
  Bottom 0.406: J6.27 150.42,107.92 151,108.5 152.86,108.5 J4.27
PB2_7
  Top 0.305: U7.3 186.5,119.48 186.5,120.12 189.5,123.12 207.5,123.12 213.38,129 213.38,133.62 209.88,137.12 172.25,137.12 164.8,129.67 J2.43 164.42,129.67 163.25,128.5 157,128.5 155.38,130.12 154.34,130.12 J4.43 154.16,130.12 153.5,130.12 152.38,129 151.12,129 150.36,128.24 J6.43
PB2_8
  Top 0.305: 211.12,151.12 210.5,150.5 189.62,150.5 186.38,147.25 186.38,146.68 U8.3 | J2.59 163.87,149.99 162.62,148.75 157.5,148.75 155.75,150.5 154.28,150.5 J4.59
  Top 0.406: J2.59 165.62,149.99 176.38,160.75 210.88,160.75 213.25,158.38 213.25,153.25 211.12,151.12 | U8.3 186.41,146.91
PB3_1
  Bottom 0.305: U2.4 31.3,58.32 30,59.62 30,63.25 30.62,63.88 34.38,63.88 36.88,61.38 41.83,61.38 RN2.4
PB3_2
  Bottom 0.305: U3.4 31.3,85.82 30,87.12 30,90.75 31.12,91.88 34.5,91.88 38.25,88.12 42.95,88.12 RN4.4
PB3_3
  Bottom 0.305: U1.4 35.8,117.69 34.5,119 34.5,123.25 35,123.75 38.5,123.75 42.25,120 45.95,120 RN6.4
PB3_4
  Bottom 0.305: U4.4 35.75,144.69 35.75,144.75 34.5,146 34.5,151.25 35.5,152.25 38.75,152.25 44.5,146.5 45.33,146.5 RN8.4
PB3_5
  Top 0.305: U5.4 187.81,65.43 188.62,66.25 189.25,66.25 194,71 210.25,71 214.5,75.25 214.5,82.62 212.62,84.5 182.25,84.5 176.5,90.25 163.32,90.25 J2.12 162.07,89 161.5,89 159.62,90.88 153.25,90.88 151.95,89.58 J4.12
  Top 0.406: C20.1 187.5,63.38 187.75,63.62 187.75,64.72 U5.4 | J10.12 121.23,87.5 123.75,87.5 125.07,88.82 J8.12 130.55,88.75 131.5,88.75 132.66,87.59 J6.12 | J13.12 123.66,162.79 124.12,163.25 128.62,163.25 129.5,164.12 130.62,164.12 131.5,163.25 132.25,163.25 J15.12 139.48,162.86 140.12,163.5 141.38,163.5 142.56,162.31 J17.12 146.81,162.31 149.75,165.25 152.75,165.25 153.88,164.12 154.56,164.12 J19.12
  Bottom 0.305: RN10.4 136.47,88.03 134.5,90 131.66,90 J8.12 | J10.12 119.75,88.63 115.75,92.62 115.75,160.5 119.25,164 121.06,164 J13.12 | J6.12 141.61,87.6 142.88,88.88 150.38,88.88 151.12,89.62 151.66,89.62 J4.12
PB3_6
  Top 0.305: J2.28 162.6,109.35 163.88,110.62 165.88,110.62 166.62,109.88 212.88,109.88 214.38,108.38 214.38,99.5 211.88,97 191.75,97 190.25,95.5 189.25,95.5 187.75,94 187.75,93.7 U6.4 | 162,109.25 157,109.25 155.12,111.12 153.62,111.12 152.25,109.75 151.86,109.75 J4.28
  Top 0.406: 162,109.25 J2.28 | C36.1 187.62,92.25 187.75,92.38 187.75,93.59 U6.4 | J10.28 120.3,108.95 121.5,107.75 123.5,107.75 124.75,109 130.34,109 J8.28 131.11,109.14 132.5,107.75 141.44,107.75 J6.28
  Bottom 0.305: RN12.4 169.85,109.03 169,109.88 166.62,109.88 165.88,110.62 163.38,110.62 J2.28
  Bottom 0.406: J6.28 141.61,108.11 142.75,109.25 151.06,109.25 J4.28
PB3_7
  Top 0.305: U7.4 187.5,119.33 187.5,120.25 187.88,120.25 190.25,122.62 207.75,122.62 214.12,129 214.12,133.88 210.25,137.75 171.88,137.75 165.12,131 164.25,131 162.92,129.67 J2.44 157.08,129.67 155.25,131.5 153,131.5 J4.44 151.62,130.12 151.12,130.12 150.5,129.5 142.75,129.5 141.61,128.36 J6.44
PB3_8
  Top 0.305: 211.38,150.5 210.88,150 190.5,150 187.75,147.25 | J2.60 157.26,149.99 155.5,151.75 152.88,151.75 152.68,151.55 152.68,151.5 J4.60
  Top 0.406: J2.60 162.37,149.99 163.5,151.12 165.75,151.12 176,161.38 211.25,161.38 214,158.62 214,153.12 211.38,150.5 | 187.75,147.25 187.75,146.72 U8.4
PB4_1
  Bottom 0.305: U2.5 31.32,57.05 29.5,58.88 29.5,63.5 30.38,64.38 34.62,64.38 37,62 41.7,62 RN2.5
PB4_2
  Bottom 0.305: U3.5 31.57,84.55 29.5,86.62 29.5,91 30.88,92.38 34.88,92.38 38.38,88.88 42.95,88.88 RN4.5
PB4_3
  Bottom 0.305: U1.5 36.08,116.42 34,118.5 34,123.5 34.75,124.25 38.75,124.25 42.25,120.75 45.95,120.75 RN6.5
PB4_4
  Bottom 0.305: RN8.5 45.38,147.25 44.5,147.25 39,152.75 35.25,152.75 34,151.5 34,145.25 35.83,143.43 U4.5
PB4_5
  Top 0.305: 189.07,64.95 U5.5 189.25,64.94 189.25,65.5 194.25,70.5 210.88,70.5 215.12,74.75 215.12,82.75 212.75,85.12 182.62,85.12 176,91.75 164.82,91.75 J2.13 164.45,91.38 163.62,91.38 162.62,90.38 161.5,90.38 159.76,92.12 J4.13
  Top 0.406: C21.1 188.75,63.75 189,64 189,64.69 U5.5 | J13.13 120.25,160.25 121.5,159 124.62,159 125.88,160.25 130.04,160.25 J15.13 130.56,160.31 131.88,159 139.5,159 140.25,159.75 140.7,159.75 J17.13 141.35,159.78 142.62,158.5 149.12,158.5 151.12,160.5 151.12,160.53 J19.13 | J10.13 122.97,91.5 123.75,91.5 124.75,92.5 131.25,92.5 132.39,91.36 J8.13 133.16,91.5 143,91.5 144.14,90.35 J6.13
  Bottom 0.305: RN10.5 137.28,88.97 134.75,91.5 133.16,91.5 J8.13 | J4.13 153.87,92.12 152.62,90.88 151.38,90.88 150.62,90.12 144.16,90.12 J6.13
  Bottom 0.406: J13.13 119.5,160.25 117.25,158 117.25,94.5 119.38,92.38 121.44,92.38 J10.13
PB4_6
  Top 0.305: U6.5 189.12,93.69 189.12,94.25 189.88,95 190.5,95 192,96.5 212.12,96.5 215.12,99.5 215.12,108.38 213,110.5 167.25,110.5 165.86,111.89 J2.29 163.89,111.89 162.75,110.75 157.5,110.75 155.75,112.5 154.31,112.5 J4.29
  Top 0.406: C37.1 189.12,93.59 U6.5 | J6.29 142.92,111.68 J8.29 132.97,111.62 132.25,111.62 131.12,112.75 124.75,112.75 123.49,111.49 J10.29
  Bottom 0.305: RN12.5 170.65,109.22 168.12,111.75 164.78,111.75 J2.29
  Bottom 0.406: J6.29 150.45,110.45 151.12,111.12 152.38,111.12 153.62,112.38 154.19,112.38 J4.29
PB4_7
  Top 0.305: U7.5 188.75,119.34 188.75,120.12 190.75,122.12 208,122.12 214.62,128.75 214.62,134.12 210.38,138.38 171,138.38 164.83,132.21 J2.45 164.21,132.21 163,131 156.88,131 155.25,132.62 154.38,132.62 J4.45 154.12,132.62 153.25,132.62 151.88,131.25 151.25,131.25 150.78,130.78 J6.45
PB4_8
  Top 0.305: 189,147.38 189.12,147.38 191.25,149.5 211.5,149.5 211.88,149.88
  Top 0.406: J2.61 165.78,152.53 175.38,162.12 211.5,162.12 214.75,158.88 214.75,152.75 211.88,149.88 | 189,147.38 189,146.69 U8.5
PB5_1
  Bottom 0.305: U2.6 31.22,55.78 29,58 29,63.88 30,64.88 35.12,64.88 37,63 41.8,63 RN2.6
PB5_2
  Bottom 0.305: U3.6 31.59,83.28 29,85.88 29,91.25 30.62,92.88 35.12,92.88 38.25,89.75 42.92,89.75 RN4.6
PB5_3
  Bottom 0.305: U1.6 36.34,115.16 33.5,118 33.5,123.75 34.5,124.75 39,124.75 42.25,121.5 45.9,121.5 RN6.6
PB5_4
  Bottom 0.305: RN8.6 45.42,148 44.5,148 39.25,153.25 35,153.25 33.5,151.75 33.5,144.75 36.09,142.16 U4.6
PB5_5
  Top 0.305: U5.6 190.34,65.47 194.75,69.88 211.12,69.88 215.75,74.5 215.75,82.88 212.88,85.75 182.88,85.75 175.75,92.88 163.41,92.88 J2.14 162.05,91.62 161.5,91.62 159.75,93.38 153.25,93.38 151.99,92.12 J4.14
  Top 0.406: 190.25,63.12 190.34,63.12 | 190.34,63.12 U5.6 | C22.1 190.12,62.91 190.34,63.12 | J13.14 124.75,160.25 126,161.5 130.88,161.5 132.06,160.31 J15.14 139.56,160.31 140.25,161 141.5,161 142.72,159.78 J17.14 147.9,159.78 150.88,162.75 153.4,162.75 J19.14 | J10.14 121.28,90 123.75,90 125.11,91.36 J8.14 130.84,91 131.25,91 132.12,90.13 J6.14
  Bottom 0.305: RN10.6 138.07,89.55 135.12,92.5 131.62,92.5 J8.14 | J13.14 121.62,160.25 120.5,161.38 119.25,161.38 116.75,158.88 116.75,93.62 119.25,91.12 120.06,91.12 J10.14 | J6.14 141.76,90.13 143,91.38 150.97,91.38 J4.14
PB5_6
  Top 0.305: J2.30 162.39,111.89 163.62,113.12 165.62,113.12 167.62,111.12 213.25,111.12 215.62,108.75 215.62,99.25 212.38,96 192.38,96 191.75,95.38 191.62,95.38 190.38,94.12 190.38,93.67 U6.6 | 162.09,111.88 157.62,111.88 155.75,113.75 153.03,113.75 J4.30
  Top 0.406: 162.09,111.88 J2.30 | C38.1 190.38,93.62 U6.6 | J10.30 120.26,111.49 121.5,110.25 123.25,110.25 124.5,111.5 130.3,111.5 J8.30 130.82,111.68 132,110.5 141.56,110.5 J6.30
  Bottom 0.305: RN12.6 171.45,109.8 168,113.25 163.47,113.25 J2.30
  Bottom 0.406: J6.30 142.2,110.45 143.5,111.75 150.38,111.75 151.12,112.5 151.64,112.5 J4.30
PB5_7
  Top 0.305: U7.6 190.25,119.42 190.25,120.25 191.62,121.62 208.25,121.62 215.25,128.62 215.25,134.5 210.75,139 170.62,139 165.12,133.5 164.38,133.5 163.08,132.21 J2.46 157.54,132.21 155.62,134.12 153.88,134.12 152.5,132.75 J4.46 150.95,132 143,132 141.78,130.78 J6.46
PB5_8
  Top 0.305: U8.6 190.22,147.09 192.12,149 212,149 212.25,149.25
  Top 0.406: J2.62 162.16,152.53 163.25,153.62 165.88,153.62 175,162.75 211.75,162.75 215.38,159.12 215.38,152.38 212.25,149.25 | 190.12,146.74 U8.6
PB6_1
  Bottom 0.305: U2.7 31.24,54.51 28.5,57.25 28.5,64 29.88,65.38 35.5,65.38 37.25,63.62 41.73,63.62 RN2.7
PB6_2
  Bottom 0.305: U3.7 31.11,82.01 28.5,84.62 28.5,91.5 30.38,93.38 35.5,93.38 38.38,90.5 RN4.7
PB6_3
  Bottom 0.305: U1.7 36.11,113.89 33,117 33,124 34.25,125.25 39.25,125.25 42.25,122.25 45.85,122.25 RN6.7
PB6_4
  Bottom 0.305: RN8.7 44.75,148.75 39.75,153.75 34.75,153.75 33,152 33,143.75 35.86,140.88 U4.7
PB6_5
  Top 0.305: U5.7 191.62,65.36 195.62,69.38 211.75,69.38 216.38,74 216.38,83 213.12,86.25 183.25,86.25 175.38,94.12 164.66,94.12 J2.15 164.53,94 163.75,94 162.5,92.75 161.62,92.75 159.72,94.66 J4.15
  Top 0.406: C23.1 191.5,64.66 U5.7 | J17.15 139.87,156.38 132.12,156.38 130.72,157.78 J15.15 130.08,157.75 125.62,157.75 124.25,156.38 121.75,156.38 120.41,157.71 J13.15 | J10.15 123.59,93.71 125,95.12 131.25,95.12 132.47,93.9 J8.15 133.12,94 143,94 144.14,92.85 J6.15
  Bottom 0.305: RN10.7 138.88,91.12 136.12,93.88 133.05,93.88 J8.15 | J4.15 153.28,94.66 152,93.38 151,93.38 150.25,92.62 144.19,92.62 J6.15
  Bottom 0.406: J13.15 119.71,157.71 118.5,156.5 118.5,96 119.62,94.88 121.48,94.88 J10.15
PB6_6
  Top 0.305: U6.7 191.62,93.66 191.62,94.25 192.88,95.5 212.75,95.5 216.25,99 216.25,109 213.62,111.62 168.12,111.62 165.32,114.43 J2.31 163.93,114.43 162.75,113.25 157.38,113.25 155.65,114.97 J4.31
  Top 0.406: C39.1 191.75,93.51 U6.7 | J10.31 123.28,114.03 124.75,115.5 131,115.5 132.28,114.22 J8.31 142.92,114.22 J6.31
  Bottom 0.305: RN12.7 172.25,110.75 168.5,114.5 164.72,114.5 J2.31
  Bottom 0.406: J6.31 150.25,113 151,113.75 152.25,113.75 153.47,114.97 J4.31
PB6_7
